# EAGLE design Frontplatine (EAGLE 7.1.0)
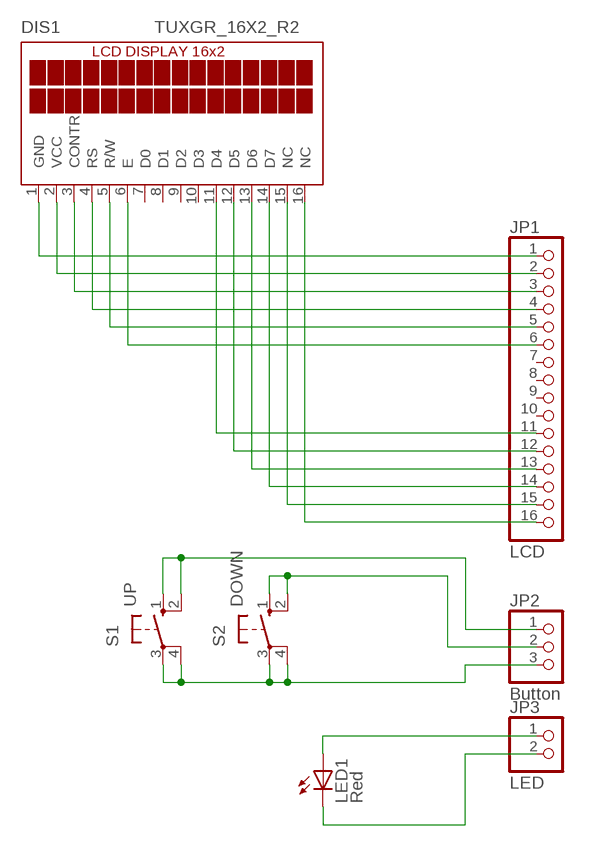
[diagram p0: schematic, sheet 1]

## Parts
DIS1  TUXGR_16X2_R2  [TUXGR_16X2_R2]
JP1  LCD  PINHD-1X16  [1X16]
JP2  Button  PINHD-1X3  [1X03]
JP3  LED  PINHD-1X2  [1X02]
LED1  Red  LED5MM  [LED5MM]
S1  UP  10-XX  [B3F-10XX]
S2  DOWN  10-XX  [B3F-10XX]

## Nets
N$1: DIS1.1(GND) JP1.1
N$2: DIS1.2(VCC) JP1.2
N$3: DIS1.3(CONTR) JP1.3
N$4: DIS1.4(RS) JP1.4
N$5: DIS1.5(R/W) JP1.5
N$6: DIS1.6(E) JP1.6
N$7: DIS1.16(NC) JP1.16
N$8: DIS1.15(NC) JP1.15
N$9: DIS1.14(D7) JP1.14
N$10: DIS1.13(D6) JP1.13
N$11: DIS1.12(D5) JP1.12
N$12: DIS1.11(D4) JP1.11
N$13: JP2.1 S1.1(S) S1.2(S1)
N$14: JP2.3 S1.3(P) S1.4(P1) S2.3(P) S2.4(P1)
N$15: JP2.2 S2.1(S) S2.2(S1)
N$16: JP3.1 LED1.A
N$17: JP3.2 LED1.K(C)
Unconnected: DIS1.7(D0) DIS1.8(D1) DIS1.9(D2) DIS1.10(D3) JP1.7 JP1.8 JP1.9 JP1.10

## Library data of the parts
DIS1 = display-lcd:TUXGR_16X2_R2: Tuxgraphics LCD display 16x2 characters reflective, without background light Source: tuxgr_12x2_r2.pdf; OC_FARNELL: unknown; OC_NEWARK: unknown
JP1 = pinhead:PINHD-1X16: PIN HEADER
JP2 = pinhead:PINHD-1X3: PIN HEADER
JP3 = pinhead:PINHD-1X2: PIN HEADER
LED1 = led:LED: LED
S1 S2 = switch-omron:10-XX: OMRON SWITCH; MPN: B3F-1000; OC_FARNELL: 176432; OC_NEWARK: 36M3542

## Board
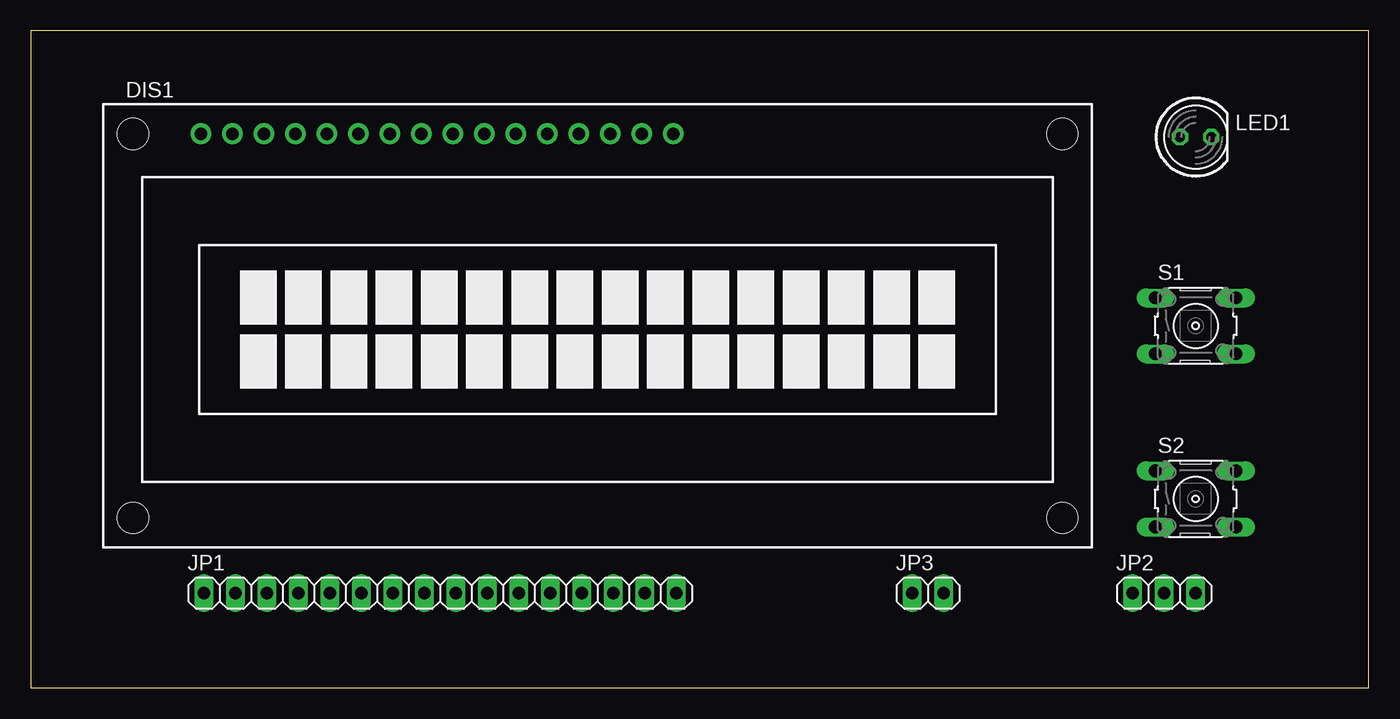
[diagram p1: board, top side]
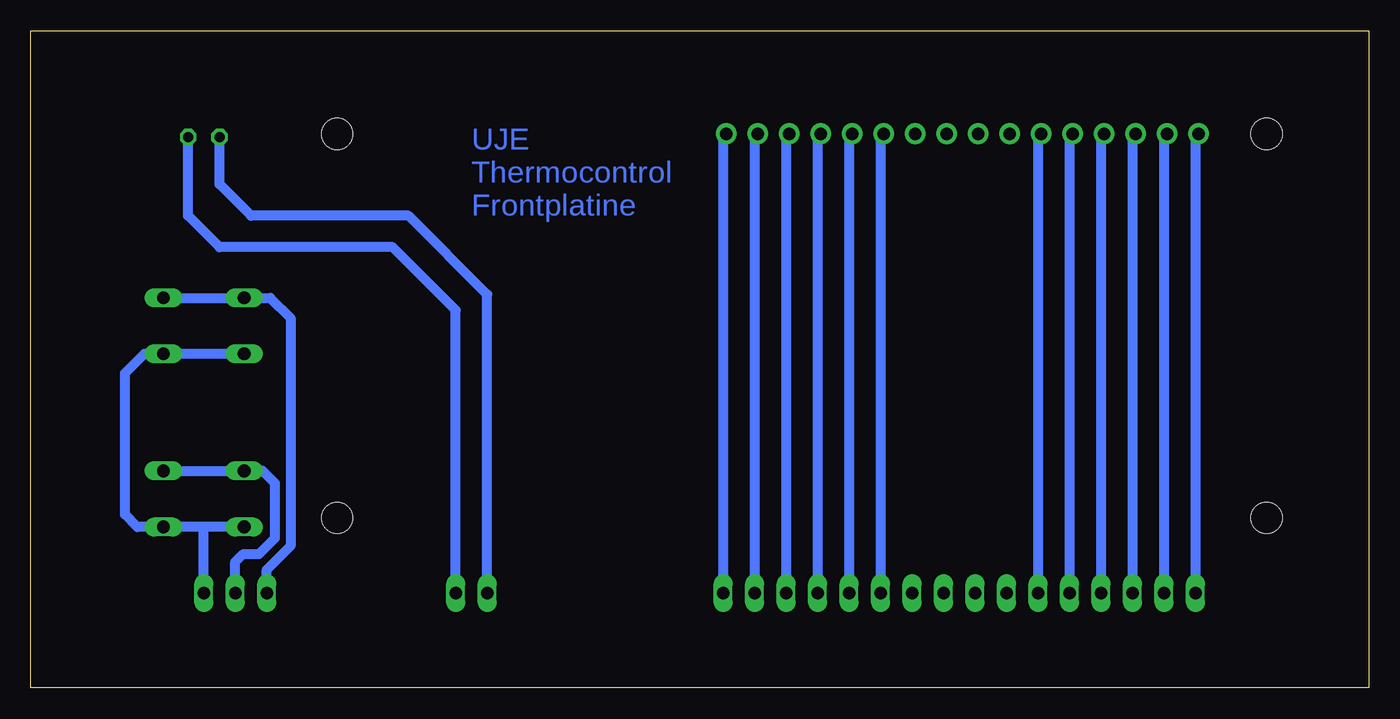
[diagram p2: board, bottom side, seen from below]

Size 107.93 x 53.01 mm. Coordinates in mm from the lower left corner, seen from the top.
Outline: 0,0 107.93,0 107.93,53.01 0,53.01 0,0
Copper layers (1*16): Top 0.035mm / dielectric 1.5mm / Bottom 0.035mm
Design rules "default": minimum track width 10mil, minimum drill 24mil, track to track 8mil, track to pad 8mil, pad to pad 8mil, via to via 8mil, smd to smd 8mil, copper to edge 40mil, drill to drill 8mil, minimum pad ring 10mil, minimum via ring 8mil, stop-mask expansion 4mil, vias tented up to drill 0mil, thermal gap 10mil

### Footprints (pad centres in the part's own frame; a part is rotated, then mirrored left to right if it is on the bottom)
TUXGR_16X2_R2 = drill 1 pad 1.676: 1 -32,15.5; 2 -29.46,15.5; 3 -26.92,15.5; 4 -24.38,15.5; 5 -21.84,15.5; 6 -19.3,15.5; 7 -16.76,15.5; 8 -14.22,15.5; 9 -11.68,15.5; 10 -9.14,15.5; 11 -6.6,15.5; 12 -4.06,15.5; 13 -1.52,15.5; 14 1.02,15.5; 15 3.56,15.5; 16 6.1,15.5 | hole 2.5: -37.5,-15.5; 37.5,-15.5; -37.5,15.5; 37.5,15.5
1X16 = drill 1.016 long: 1 -19.05,0; 2 -16.51,0; 3 -13.97,0; 4 -11.43,0; 5 -8.89,0; 6 -6.35,0; 7 -3.81,0; 8 -1.27,0; 9 1.27,0; 10 3.81,0; 11 6.35,0; 12 8.89,0; 13 11.43,0; 14 13.97,0; 15 16.51,0; 16 19.05,0
1X03 = drill 1.016 long: 1 -2.54,0; 2 0,0; 3 2.54,0
1X02 = drill 1.016 long: 1 -1.27,0; 2 1.27,0
LED5MM = drill 0.813 octagon: A -1.27,0; K 1.27,0
B3F-10XX = drill 1.016 long: 1 -3.251,2.261; 2 3.251,2.261; 3 -3.251,-2.261; 4 3.251,-2.261

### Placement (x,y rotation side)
DIS1  45.72,29.21 0 top
JP1  33.02,7.62 0 top
JP2  91.44,7.62 0 top
JP3  72.39,7.62 0 top
LED1  93.98,44.45 0 top
S1  93.98,29.21 0 top
S2  93.98,15.24 0 top

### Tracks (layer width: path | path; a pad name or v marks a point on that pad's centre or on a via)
N$1
  Bottom 0.813: DIS1.1 13.97,44.71 JP1.1
N$2
  Bottom 0.813: DIS1.2 16.51,44.71 JP1.2
N$3
  Bottom 0.813: DIS1.3 19.05,44.71 JP1.3
N$4
  Bottom 0.813: DIS1.4 21.59,44.71 JP1.4
N$5
  Bottom 0.813: DIS1.5 24.13,44.71 JP1.5
N$6
  Bottom 0.813: DIS1.6 26.67,44.71 JP1.6
N$7
  Bottom 0.813: DIS1.16 52.07,44.71 JP1.16
N$8
  Bottom 0.813: DIS1.15 49.53,44.71 JP1.15
N$9
  Bottom 0.813: DIS1.14 46.99,44.71 JP1.14
N$10
  Bottom 0.813: DIS1.13 44.45,44.71 JP1.13
N$11
  Bottom 0.813: DIS1.12 41.91,44.71 JP1.12
N$12
  Bottom 0.813: DIS1.11 39.37,44.71 JP1.11
N$13
  Bottom 0.813: JP2.1 88.9,9.52 87,11.43 87,29.84 88.62,31.47 S1.1 S1.2
N$14
  Bottom 0.813: S1.3 S1.4 98.78,26.95 100.33,25.4 100.33,13.97 99.34,12.98 S2.4 | S2.3 93.98,12.98 | 93.98,12.98 S2.4 | S2.4 97.51,12.98 97.79,12.7 | JP2.3 93.98,12.98
N$15
  Bottom 0.813: JP2.2 91.44,10.16 90.81,10.79 89.53,10.79 88.27,12.06 88.27,16.51 89.26,17.5 S2.1 S2.2
N$16
  Bottom 0.813: JP3.1 71.12,31.75 77.47,38.1 90.17,38.1 92.71,40.64 LED1.A
N$17
  Bottom 0.813: JP3.2 73.66,30.48 78.74,35.56 92.71,35.56 95.25,38.1 LED1.K

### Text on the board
Bottom: UJE / Thermocontrol / Frontplatine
